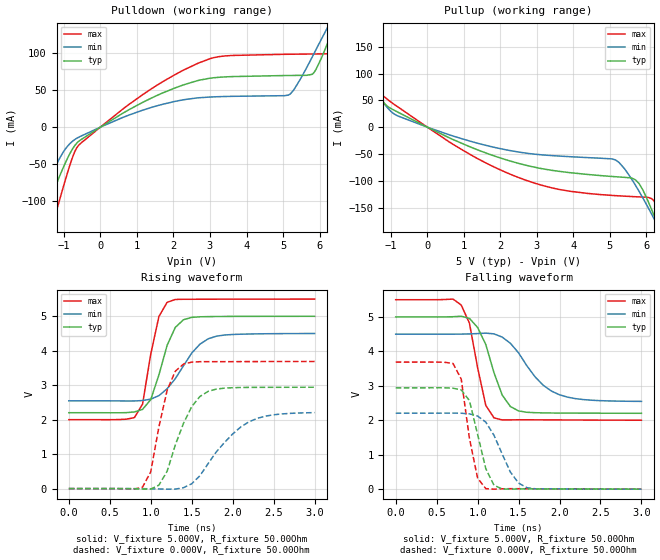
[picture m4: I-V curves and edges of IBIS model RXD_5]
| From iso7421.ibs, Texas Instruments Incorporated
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|   RXD_5 MODEL
[Model]   RXD_5
Model_type   Output
| Signals   RXD
Vmeas = 1.55V   |Reference voltage for timing measurements
Cref = 15pF   |Timing specification test load capacitance value
| variable   typ   min   max
|   (nom PVT)   (slow PVT)   (fast PVT)
|C_comp Average
C_comp   2.2969pF   2.0172pF   2.7619pF
|C_comp Output Low
|C_comp   2.4013pF   2.1415pF   2.8615pF
|C_comp Output High
|C_comp   2.1925pF   1.8929pF   2.6624pF
|   typ   min   max
[Voltage Range]   5.0V   4.5V   5.5V
[Temperature Range]   27.0   136.0   -40.0
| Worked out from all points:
|   slope of the pulldown table from 0 to 0.75 V, typ, clamps not added: 33.1 ohm
|   slope of the pullup table from 0 to 0.75 V, typ, clamps not added: 30.6 ohm
|   falling waveform, V_fixture 5.000V, R_fixture 50.00Ohm: 20-80 % time 244ps typ, 402ps min, 174ps max; typ from 5 V to 2.2 V
|   rising waveform, V_fixture 5.000V, R_fixture 50.00Ohm: 20-80 % time 229ps typ, 355ps min, 165ps max; typ from 2.2 V to 5 V
|   rising waveform, V_fixture 0.000V, R_fixture 50.00Ohm: 20-80 % time 283ps typ, 468ps min, 199ps max; typ from 0 V to 2.94 V
|   falling waveform, V_fixture 0.000V, R_fixture 50.00Ohm: 20-80 % time 179ps typ, 270ps min, 149ps max; typ from 2.94 V to 0 V
[Pulldown]
|   Voltage   I(typ)   I(min)   I(max)
-5V       -714.5mA   -538.9mA   -874.4mA
-1.9V     -193.1mA   -134.8mA   -254.5mA
-1.6V     -139.1mA   -96.57mA   -187mA
-1.4V     -105.2mA   -72.58mA   -148.9mA
-600mV    -19.52mA   -13.85mA   -24.84mA
1.4V      39.45mA    26.74mA    52.02mA
3V        66.31mA    40.77mA    92.7mA
5.15V     69.95mA    43.46mA    98.71mA
5.8V      71.58mA    95.09mA    99.05mA
6.3V      123.3mA    142.6mA    99.39mA
6.75V     177.6mA    181.7mA    143mA
10V       393.9mA    335.4mA    459mA
[Pullup]
|   Voltage   I(typ)   I(min)   I(max)
-5V       299mA      263.9mA    343.9mA
-2.95V    218.1mA    187.7mA    258.2mA
-2.3V     165.5mA    142.8mA    195.7mA
-1.35V    62.46mA    58.99mA    68.06mA
-1.05V    37.08mA    33.2mA     49.74mA
2.5V      -67.65mA   -46.46mA   -94.07mA
5.15V     -92.54mA   -61.08mA   -127.8mA
5.8V      -105.5mA   -120.1mA   -130.2mA
6.15V     -155.3mA   -163.4mA   -133.8mA
6.4V      -198.6mA   -196.3mA   -161.6mA
6.55V     -225.8mA   -216.5mA   -188.1mA
10V       -821.8mA   -667.2mA   -926.4mA
[Ramp]
R_load = 50.00Ohm
|   typ   min   max
dV/dt_r   1.765V/283.433ps   1.323V/467.725ps   2.214V/198.663ps
dV/dt_f   1.679V/244.269ps   1.171V/402.291ps   2.100V/173.620ps
[Falling Waveform]
V_fixture = 5.000V
V_fixture_min = 4.500V
V_fixture_max = 5.500V
R_fixture = 50.00Ohm
|   Time   V(typ)   V(min)   V(max)
0s        5V         4.5V       5.5V
800ps     5.021V     4.502V     5.344V
900ps     4.959V     4.507V     4.821V
1ns       4.694V     4.517V     3.526V
1.1ns     4.198V     4.53V      2.429V
1.2ns     3.38V      4.509V     2.07V
1.3ns     2.732V     4.415V     2.01V
1.5ns     2.271V     3.956V     2.014V
2ns       2.209V     2.739V     2.009V
3ns       2.202V     2.548V     2.001V
[Rising Waveform]
V_fixture = 5.000V
V_fixture_min = 4.500V
V_fixture_max = 5.500V
R_fixture = 50.00Ohm
|   Time   V(typ)   V(min)   V(max)
0s        2.202V     2.548V     2.001V
800ps     2.224V     2.543V     2.059V
900ps     2.299V     2.555V     2.452V
1ns       2.582V     2.596V     3.901V
1.1ns     3.302V     2.697V     4.995V
1.2ns     4.158V     2.897V     5.405V
1.3ns     4.679V     3.191V     5.488V
1.4ns     4.9V       3.566V     5.494V
1.7ns     4.99V      4.345V     5.496V
3ns       5V         4.5V       5.5V
[Rising Waveform]
V_fixture = 0.000V
V_fixture_min = 0.000V
V_fixture_max = 0.000V
R_fixture = 50.00Ohm
|   Time   V(typ)   V(min)   V(max)
0s        486.1pV    899.5pV    557.2pV
900ps     -11.73mV   -1.759mV   40.23mV
1ns       -15.75mV   -4.943mV   488.8mV
1.2ns     502.3mV    -16.13mV   2.853V
1.3ns     1.267V     -15mV      3.407V
1.4ns     1.893V     26.77mV    3.613V
1.5ns     2.379V     141.2mV    3.67V
1.7ns     2.821V     723mV      3.685V
2.2ns     2.937V     1.94V      3.686V
3ns       2.941V     2.205V     3.689V
[Falling Waveform]
V_fixture = 0.000V
V_fixture_min = 0.000V
V_fixture_max = 0.000V
R_fixture = 50.00Ohm
|   Time   V(typ)   V(min)   V(max)
0s        2.941V     2.205V     3.689V
700ps     2.931V     2.208V     3.648V
800ps     2.879V     2.204V     3.196V
900ps     2.573V     2.186V     1.478V
1ns       1.59V      2.123V     315.7mV
1.1ns     592.7mV    1.945V     14.54mV
1.2ns     112mV      1.563V     -1.074mV
1.4ns     553.8uV    495.8mV    12.97mV
1.6ns     7.283mV    43.36mV    11.1mV
3ns       486.1pV    899.5pV    557.2pV
